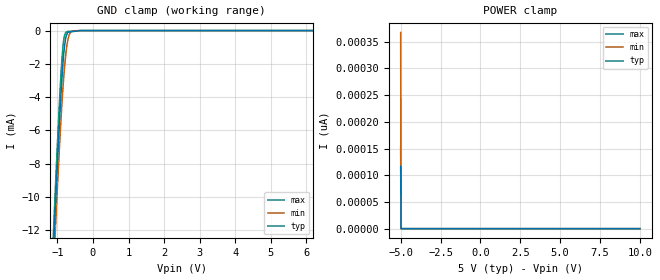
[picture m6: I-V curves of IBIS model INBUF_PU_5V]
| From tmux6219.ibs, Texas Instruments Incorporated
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| Model7
[Model]   INBUF_PU_5V
Model_type   Input
Vinl = 0.8
Vinh = 1.3
|   typ   min   max
C_comp   1.85pF   1.7pF   2.1pF
[Voltage Range]   5   4.5   5.5
[Temperature Range]   27   125   -40
[Power Clamp Reference]   5   4.5   5.5
[GND Clamp Reference]   0   0   0
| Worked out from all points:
|   GND clamp passes 1 mA (typ) near -0.80 V on its own axis
[GND Clamp]
|   Voltage   I(typ)   I(min)   I(max)
-5V       -219.2mA   -219.2mA   -219.1mA
-1.13V    -14.1mA    -15.41mA   -13.07mA
-1.04V    -9.827mA   -11.25mA   -8.704mA
-920mV    -4.606mA   -6.15mA    -3.408mA
-875mV    -2.952mA   -4.471mA   -1.814mA
-830mV    -1.615mA   -3.053mA   -700.2uA
-800mV    -957.4uA   -2.208mA   -298.3uA
-755mV    -344uA     -1.251mA   -89.41uA
-710mV    -100.8uA   -619.1uA   -51.59uA
-635mV    -79.1uA    -115.8uA   -40.66uA
-455mV    -27.09uA   -4.639uA   -14.43uA
10V       0A         0A         0A
[POWER Clamp]
|   Voltage   I(typ)   I(min)   I(max)
-5V       116.5pA    367.4pA    152.9pA
-4.97V    0A         0A         0A
-4.955V   0A         0A         0A
10V       0A         0A         0A
